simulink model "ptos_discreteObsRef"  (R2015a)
settings: Solver=ode45  StartTime=0.0  StopTime=trun  FixedStep=dt  MinStep=dt/100  RelTol=1e-12
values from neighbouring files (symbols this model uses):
  A = sys.a    [fig2_plot_FTO_REF.m]    (also in fig4_ptosref_udot.m; fig6_7_plotdata_REF.m = ptosParams.A)
  Az = ptosParams.Az    [fig6_7_plotdata_REF.m]
  B = sys.b    [fig2_plot_FTO_REF.m]    (also in fig4_ptosref_udot.m; fig6_7_plotdata_REF.m = ptosParams.B)
  Bz = ptosParams.Bz    [fig6_7_plotdata_REF.m]
  C = sys.c    [fig2_plot_FTO_REF.m]    (also in fig6_7_plotdata_REF.m = ptosParams.C; highQ_passive.m = 4.7e-07)
  c = bo/w^2    [fig2_plot_FTO_REF.m]    (also in fig4_ptosref_udot.m; fig6_7_plotdata_REF.m = ptosParams.c; fig1_motivate_ptos.m = 4.59233914625; f_ptos.m = ptosParams.c)
  cbar_min = ptosParams.cbar_min    [fig6_7_plotdata_REF.m]    (also in fptosref.m)
  cbar_plus = ptosParams.cbar_plus    [fig6_7_plotdata_REF.m]    (also in fptosref.m)
  Cz = ptosParams.Cz    [fig6_7_plotdata_REF.m]
  k2 = crossing(udot_min)    [fig4_ptosref_udot.m]    (also in fig6_7_plotdata_REF.m = ptosParams.k2; fig1_motivate_ptos.m = sqrt(2*c*alpha*xl-alpha*xl^2)/(alpha*w*c*xl); switching_curves_comp_func.m = sqrt(2*c*alpha*xl-alpha*xl^2)/(alpha*w*c*xl); ptosDampRef.m = max(abs(k2_plus), abs(k2_min)))
  k2_min = ptosParams.k2_min    [fig6_7_plotdata_REF.m]    (also in fptosref.m; ptosDampRef.m = 1/(Fxl_min - xell_min*Df_xl_plus))
  k2_plus = ptosParams.k2_plus    [fig6_7_plotdata_REF.m]    (also in fptosref.m; ptosDampRef.m = 1/(Fxl_plus - xell_plus*Df_xl_plus))
  L = ptosParams.L    [fig6_7_plotdata_REF.m]    (also in highQ_passive.m = 0.1)
  Mmin = k1_min/k2_min    [fig6_7_plotdata_REF.m]    (also in fptosref.m = ptosParams.Mmin)
  Ts = ptosParams.Ts    [fig6_7_plotdata_REF.m]
  TT = 1    [fig2_plot_FTO_REF.m]    (also in fig6_7_plotdata_REF.m = ptosParams.TT; f_ptos.m = ptosParams.TT)
  umax = 1 - x1r/c    [fig2_plot_FTO_REF.m]    (also in fig4_ptosref_udot.m; fig6_7_plotdata_REF.m = ptosParams.umax)
  umin = -1 - x1r/c    [fig2_plot_FTO_REF.m]    (also in fig4_ptosref_udot.m; fig6_7_plotdata_REF.m = ptosParams.umin)
  w = sqrt(-A(2,1))    [fig2_plot_FTO_REF.m]    (also in fig4_ptosref_udot.m; fig6_7_plotdata_REF.m = ptosParams.w; fig1_motivate_ptos.m = 1994.91133503; fptosref.m = ptosParams.w)
  X0 = [y(1), vhat(1)]'    [fig6_7_plotdata_REF.m]
  x1r = -0.4*c    [fig2_plot_FTO_REF.m]    (also in fig4_ptosref_udot.m = -0.5*c; fig6_7_plotdata_REF.m = ptosParams.x1r)
  xell_min = ptosParams.xell_min    [fig6_7_plotdata_REF.m]    (also in fptosref.m; ptosDampRef.m = wp*e1(1))
  xell_plus = ptosParams.xell_plus    [fig6_7_plotdata_REF.m]    (also in fptosref.m; ptosDampRef.m = wp*e2(1))

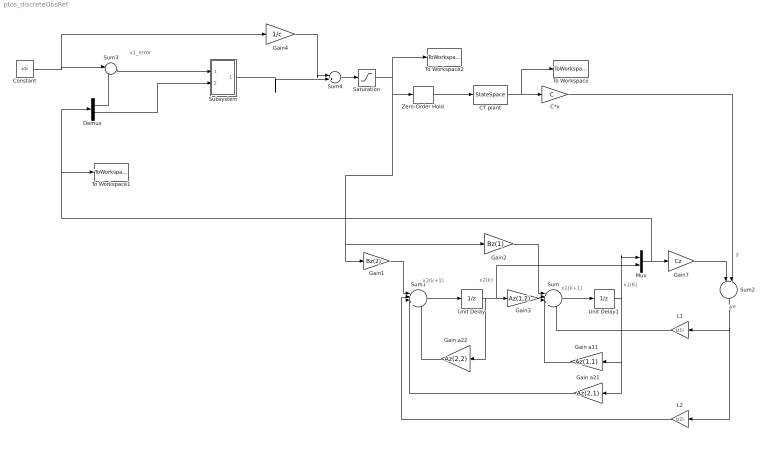
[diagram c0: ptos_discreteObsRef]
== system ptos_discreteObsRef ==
  note: x1_error
  note: y
  note: ye
  note: x2(k+1)
  note: x2(k)
  note: x1(K)
  note: x1(k+1)
  C*x : Gain  Gain=C  Multiplication=Matrix(K*u)
  CT plant : StateSpace  A=A  B=B  C=eye(2)  D=[0;0]  X0=X0
  Constant : Constant  Value=x1r
  Demux : Demux  Outputs=2
  Gain a11 : Gain  Gain=Az(1,1)
  Gain a21 : Gain  Gain=Az(2,1)
  Gain a22 : Gain  Gain=Az(2,2)
  Gain1 : Gain  Gain=Bz(2)
  Gain2 : Gain  Gain=Bz(1)
  Gain3 : Gain  Gain=Az(1,2)
  Gain4 : Gain  Gain=1/c
  Gain7 : Gain  Gain=Cz  Multiplication=Matrix(K*u)
  L1 : Gain  Gain=L(1)
  L2 : Gain  Gain=L(2)
  Mux : Mux  Inputs=2
  Saturation : Saturate  UpperLimit=TT  LowerLimit=-TT
  Subsystem : Subsystem
  Sum : Sum  Inputs=|++++
  Sum1 : Sum  Inputs=|++++
  Sum2 : Sum  Inputs=|-+
  Sum3 : Sum  Inputs=|-+
  Sum4 : Sum  Inputs=|++
  To Workspace : ToWorkspace  VariableName=xplant  SaveFormat=Timeseries  SampleTime=Ts
  To Workspace1 : ToWorkspace  VariableName=xhat  SaveFormat=Timeseries  SampleTime=Ts
  To Workspace2 : ToWorkspace  VariableName=uptos  SaveFormat=Timeseries  SampleTime=Ts
  Unit Delay : UnitDelay  InitialCondition=X0(2)  SampleTime=Ts
  Unit Delay1 : UnitDelay  InitialCondition=X0(1)  SampleTime=Ts
  Zero-Order Hold : ZeroOrderHold  SampleTime=Ts
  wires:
  Sum/1 -> Unit Delay1/1
  Unit Delay1/1 -> Gain a21/1, Gain a11/1, Mux/1
  Gain2/1 -> Sum/1
  Sum1/1 -> Unit Delay/1
  Gain1/1 -> Sum1/1
  Gain3/1 -> Sum/2
  Unit Delay/1 -> Gain a22/1, Mux/2, Gain3/1
  Gain a21/1 -> Sum1/3
  Gain a22/1 -> Sum1/4
  CT plant/1 -> To Workspace/1, C*x/1
  Gain a11/1 -> Sum/3
  Gain7/1 -> Sum2/1
  Sum2/1 -> L2/1, L1/1
  L1/1 -> Sum/4
  L2/1 -> Sum1/2
  Zero-Order Hold/1 -> CT plant/1
  C*x/1 -> Sum2/2
  Constant/1 -> Gain4/1, Sum3/1
  Gain4/1 -> Sum4/1
  Subsystem/1(u(k)) -> Sum4/2
  Sum3/1 -> Subsystem/1(x1e)
  Demux/1 -> Sum3/2
  Demux/2 -> Subsystem/2(x2)
  Mux/1 -> To Workspace1/1, Demux/1, Gain7/1
  Sum4/1 -> Saturation/1
  Saturation/1 -> Gain1/1, Gain2/1, Zero-Order Hold/1, To Workspace2/1

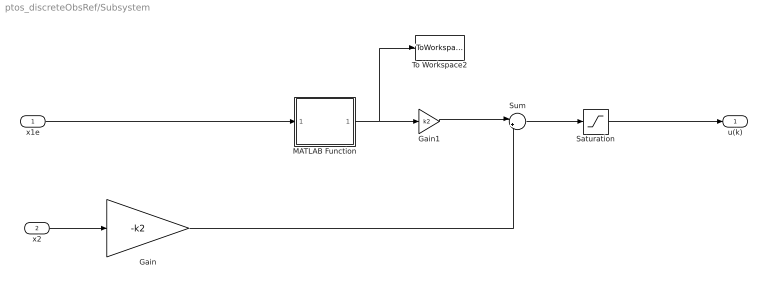
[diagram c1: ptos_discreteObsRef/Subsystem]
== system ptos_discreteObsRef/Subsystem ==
  x1e : Inport
  x2 : Inport  Port=2
  Gain : Gain  Gain=-k2
  Gain1 : Gain  Gain=k2
  MATLAB Function : MATLAB Function  TreatAsAtomicUnit=on
  Saturation : Saturate  UpperLimit=umax  LowerLimit=-abs(umin)
  Sum : Sum  Inputs=|++
  To Workspace2 : ToWorkspace  VariableName=fptos  SaveFormat=Timeseries  SampleTime=Ts
  u(k) : Outport
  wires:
  x2/1 -> Gain/1
  MATLAB Function/1(fp) -> To Workspace2/1, Gain1/1
  Gain1/1 -> Sum/1
  Gain/1 -> Sum/2
  Sum/1 -> Saturation/1
  Saturation/1 -> u(k)/1
  x1e/1 -> MATLAB Function/1(x1e)

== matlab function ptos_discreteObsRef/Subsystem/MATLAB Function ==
function fp = fptosref(x1e, xell_min, xell_plus, k2_min, k2_plus, Mmin, cbar_min, cbar_plus, w)
%#codegen


if (x1e < -abs(xell_min))
   fp =  w*sqrt(2*cbar_min*abs(x1e) -x1e.^2) - 1/k2_min;
elseif(x1e > -abs(xell_min) && x1e < xell_plus );
    fp   = -Mmin*x1e;
else (x1e >= xell_plus);
    fp = -w*sqrt(2*cbar_plus*x1e -x1e.^2) + 1/k2_plus;
end


fp = fp;
